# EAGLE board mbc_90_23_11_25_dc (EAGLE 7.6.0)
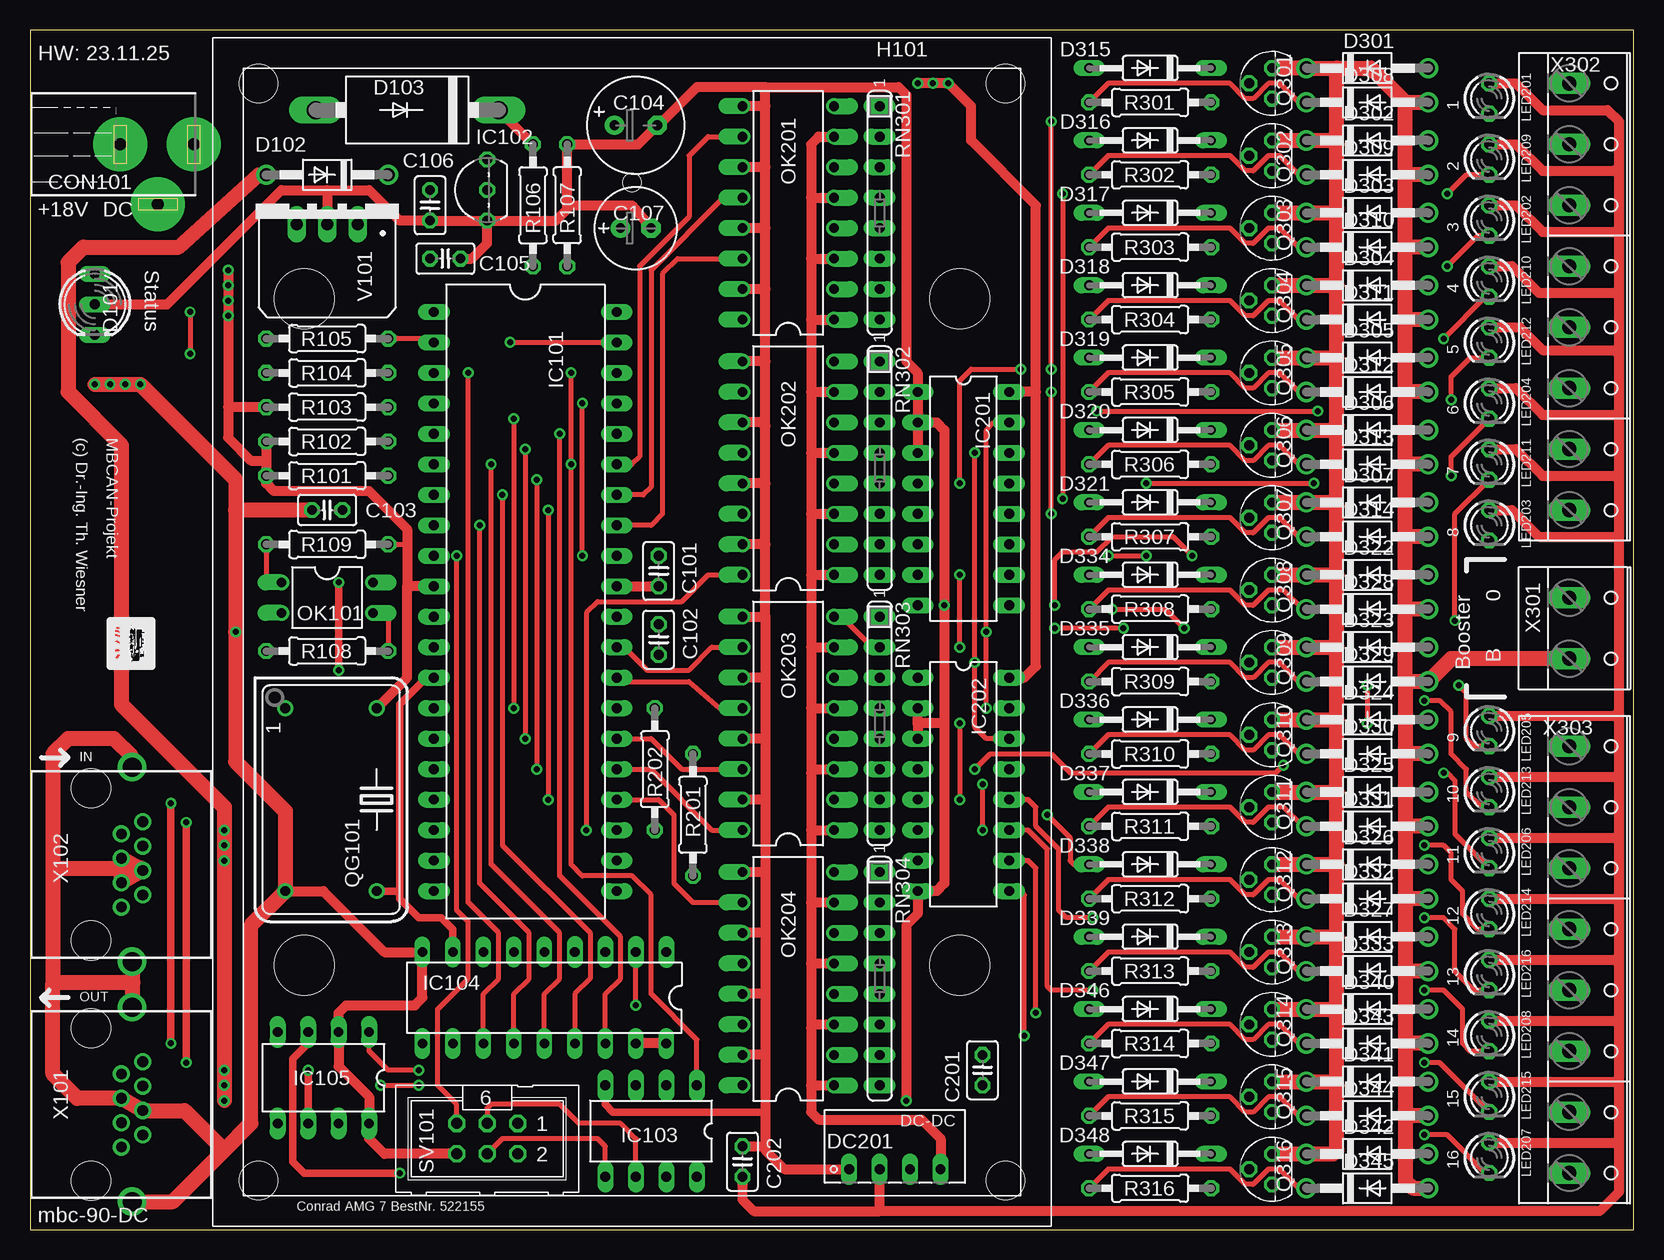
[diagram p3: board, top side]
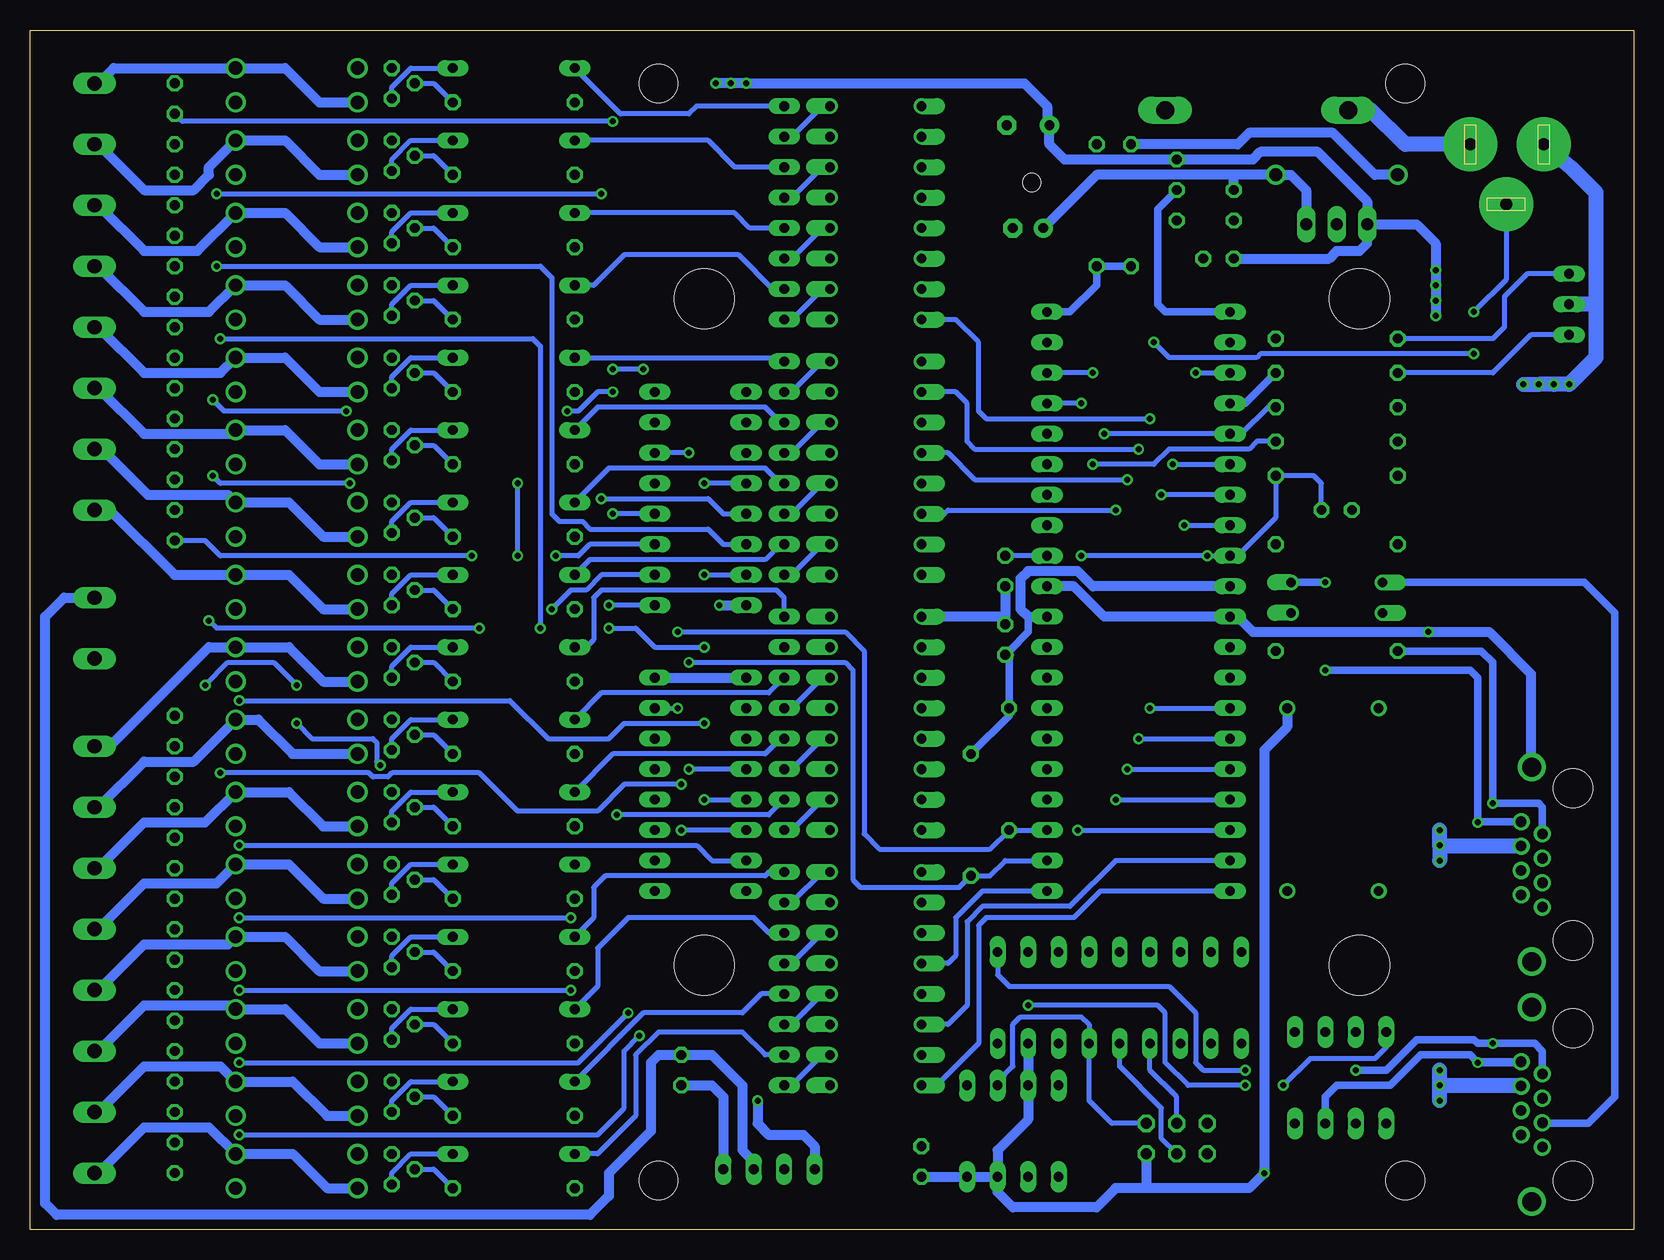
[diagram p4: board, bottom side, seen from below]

Size 133.66 x 99.99 mm. Coordinates in mm from the lower left corner, seen from the top.
Outline: 0,99.99 0,0 133.66,0 133.66,99.99 0,99.99
Copper layers (1*16): Top 0.035mm / dielectric 1.5mm / Bottom 0.035mm
Design rules "default *": minimum track width 10mil, minimum drill 0.5mm, track to track 8mil, track to pad 8mil, pad to pad 8mil, via to via 8mil, smd to smd 8mil, copper to edge 40mil, drill to drill 8mil, minimum pad ring 10mil, minimum via ring 8mil, stop-mask expansion 4mil, vias tented up to drill 0mil, thermal gap 10mil

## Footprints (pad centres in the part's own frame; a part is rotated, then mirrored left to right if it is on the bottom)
C025-025X050 = drill 0.813 octagon: 1 -1.27,0; 2 1.27,0
E3,5-8 = drill 0.813 pad 1.6: + -1.778,0 | drill 0.813 pad 1.6 octagon: - 1.778,0
E2,5-7 = drill 0.813 pad 1.6: + -1.27,0 | drill 0.813 pad 1.6 octagon: - 1.27,0
POWER-JACK = drill 1 pad 4.5: 1 0,6.03; 2 0,-0.12; 3 5,3.03
DUOLED5MM = drill 0.813 long: AG -2.54,0; AR 2.54,0; K 0,0
DO41-10 = drill 1.118: A 5.08,0; C -5.08,0
DO201-15 = drill 1.499 long: A 7.62,0; C -7.62,0
DO35-10 = drill 0.813 long: A 5.08,0; C -5.08,0
NME = drill 0.813 long: 1 0,3.81; 2 0,1.27; 3 0,-1.27; 4 0,-3.81
MODULGEHÄUSE-1 = hole 3.2: -45.72,-31.115; -45.72,31.115; 45.72,31.115; 45.72,-31.115 | hole 5: -27.781,-27.305; 27.781,-27.305; -27.781,27.305; 27.781,27.305 | hole 1.5: -37.465,0
DIL40 = drill 0.813 long: 1 -24.13,-7.62; 2 -21.59,-7.62; 3 -19.05,-7.62; 4 -16.51,-7.62; 5 -13.97,-7.62; 6 -11.43,-7.62; 7 -8.89,-7.62; 8 -6.35,-7.62; 9 -3.81,-7.62; 10 -1.27,-7.62; 11 1.27,-7.62; 12 3.81,-7.62; 13 6.35,-7.62; 14 8.89,-7.62; 15 11.43,-7.62; 16 13.97,-7.62; 17 16.51,-7.62; 18 19.05,-7.62; 19 21.59,-7.62; 20 24.13,-7.62; 21 24.13,7.62; 22 21.59,7.62; 23 19.05,7.62; 24 16.51,7.62; 25 13.97,7.62; 26 11.43,7.62; 27 8.89,7.62; 28 6.35,7.62; 29 3.81,7.62; 30 1.27,7.62; 31 -1.27,7.62; 32 -3.81,7.62; 33 -6.35,7.62; 34 -8.89,7.62; 35 -11.43,7.62; 36 -13.97,7.62; 37 -16.51,7.62; 38 -19.05,7.62; 39 -21.59,7.62; 40 -24.13,7.62
TO92- = drill 0.813 octagon: 1 -2.54,0; 2 0,0; 3 2.54,0
DIL8 = drill 0.813 long: 1 -3.81,-3.81; 2 -1.27,-3.81; 3 1.27,-3.81; 4 3.81,-3.81; 5 3.81,3.81; 6 1.27,3.81; 7 -1.27,3.81; 8 -3.81,3.81
DIL18 = drill 0.813 long: 1 -10.16,-3.81; 2 -7.62,-3.81; 3 -5.08,-3.81; 4 -2.54,-3.81 | drill 0.8 long: 5 0,-3.81; 6 2.54,-3.81; 7 5.08,-3.81; 8 7.62,-3.81; 9 10.16,-3.81; 10 10.16,3.81; 11 7.62,3.81; 12 5.08,3.81; 13 2.54,3.81; 14 0,3.81; 15 -2.54,3.81; 16 -5.08,3.81; 17 -7.62,3.81; 18 -10.16,3.81
DIL08 = drill 0.813 long: 1 -3.81,-3.81; 2 -1.27,-3.81; 3 1.27,-3.81; 4 3.81,-3.81; 5 3.81,3.81; 6 1.27,3.81; 7 -1.27,3.81; 8 -3.81,3.81
DIL16 = drill 0.813 long: 1 -8.89,-3.81; 2 -6.35,-3.81; 3 -3.81,-3.81; 4 -1.27,-3.81; 5 1.27,-3.81; 6 3.81,-3.81; 7 6.35,-3.81; 8 8.89,-3.81; 9 8.89,3.81; 10 6.35,3.81; 11 3.81,3.81; 12 1.27,3.81; 13 -1.27,3.81; 14 -3.81,3.81; 15 -6.35,3.81; 16 -8.89,3.81
LED3MM = drill 0.813 octagon: A -1.27,0; K 1.27,0
DIL04 = drill 0.813 offset: 1 -1.27,-3.81; 2 1.27,-3.81; 3 1.27,3.81; 4 -1.27,3.81
DIL16' = drill 0.813 offset: 1 -8.89,-3.81; 2 -6.35,-3.81; 3 -3.81,-3.81; 4 -1.27,-3.81; 5 1.27,-3.81; 6 3.81,-3.81; 7 6.35,-3.81; 8 8.89,-3.81; 9 8.89,3.81; 10 6.35,3.81; 11 3.81,3.81; 12 1.27,3.81; 13 -1.27,3.81; 14 -3.81,3.81; 15 -6.35,3.81; 16 -8.89,3.81
TO92 = drill 0.813 octagon: 1 1.27,0; 2 0,1.905; 3 -1.27,0
DIL14S = drill 0.813: 1 -7.62,-3.81; 7 7.62,-3.81; 8 7.62,3.81; 14 -7.62,3.81
0207/10 = drill 0.813 octagon: 1 -5.08,0; 2 5.08,0
SIL8 = drill 0.813 long: 1 -8.89,0; 2 -6.35,0; 3 -3.81,0; 4 -1.27,0; 5 1.27,0; 6 3.81,0; 7 6.35,0; 8 8.89,0
ML6 = drill 0.914 octagon: 1 -2.54,-1.27; 2 -2.54,1.27; 3 0,-1.27; 4 0,1.27; 5 2.54,-1.27; 6 2.54,1.27
TRACO-TSR-1 = drill 1.016 long: GND 0,2.54; IN -2.54,2.54; OUT 2.54,2.54
0446200002 = drill 0.889 pad 1.422: 1 3.556,2.54; 2 2.54,4.318; 3 1.524,2.54; 4 0.508,4.318; 5 -0.508,2.54; 6 -1.524,4.318; 7 -2.54,2.54; 8 -3.556,4.318 | drill 1.575 pad 2.286: S@1 -8.103,3.429; S@2 8.103,3.429 | hole 3.251: 6.35,0; -6.35,0
W237-132 = drill 1.194 long: 1 -2.54,-0.635; 2 2.54,-0.635
W237-8P = drill 1.194 long: 1 -17.78,-0.635; 2 -12.7,-0.635; 3 -7.62,-0.635; 4 -2.54,-0.635; 5 2.54,-0.635; 6 7.62,-0.635; 7 12.7,-0.635; 8 17.78,-0.635

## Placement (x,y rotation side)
C101  100n  [C025-025X050]  52.39,54.91 270 top
C102  100n  [C025-025X050]  52.39,49.19 90 top
C103  100n  [C025-025X050]  24.77,59.99 180 top
C104  470u/16V  [E3,5-8]  50.48,92.06 0 top
C105  100n  [C025-025X050]  34.61,80.94 0 top
C106  100n  [C025-025X050]  33.34,85.39 270 top
C107  47u/35V  [E2,5-7]  50.48,83.48 0 top
C201  100n  [C025-025X050]  79.38,13.32 90 top
C202  100n  [C025-025X050]  59.37,5.7 90 top
CON101  [POWER-JACK]  7.62,90.47 270 top
D101  Status  [DUOLED5MM]  5.4,77.13 270 top
D102  1N4004  [DO41-10]  24.77,87.93 180 top
D103  1N5400  [DO201-15]  31.43,93.33 180 top
D301  1N4001  [DO41-10]  111.44,96.82 0 top
D302  1N4001  [DO41-10]  111.44,90.79 0 top
D303  1N4001  [DO41-10]  111.44,84.75 0 top
D304  1N4001  [DO41-10]  111.44,78.72 0 top
D305  1N4001  [DO41-10]  111.44,72.69 0 top
D306  1N4001  [DO41-10]  111.44,66.66 0 top
D307  1N4001  [DO41-10]  111.44,60.62 0 top
D308  1N4001  [DO41-10]  111.44,93.96 0 top
D309  1N4001  [DO41-10]  111.44,87.93 0 top
D310  1N4001  [DO41-10]  111.44,81.9 0 top
D311  1N4001  [DO41-10]  111.44,75.86 0 top
D312  1N4001  [DO41-10]  111.44,69.83 0 top
D313  1N4001  [DO41-10]  111.44,63.8 0 top
D314  1N4001  [DO41-10]  111.44,57.76 0 top
D315  1N4148  [DO35-10]  93.34,96.82 180 top
D316  1N4148  [DO35-10]  93.34,90.79 180 top
D317  1N4148  [DO35-10]  93.34,84.75 180 top
D318  1N4148  [DO35-10]  93.34,78.72 180 top
D319  1N4148  [DO35-10]  93.34,72.69 180 top
D320  1N4148  [DO35-10]  93.34,66.66 180 top
D321  1N4148  [DO35-10]  93.34,60.62 180 top
D322  1N4001  [DO41-10]  111.44,54.59 0 top
D323  1N4001  [DO41-10]  111.44,48.56 0 top
D324  1N4001  [DO41-10]  111.44,42.52 0 top
D325  1N4001  [DO41-10]  111.44,36.49 0 top
D326  1N4001  [DO41-10]  111.44,30.46 0 top
D327  1N4001  [DO41-10]  111.44,24.43 0 top
D328  1N4001  [DO41-10]  111.44,51.73 0 top
D329  1N4001  [DO41-10]  111.44,45.7 0 top
D330  1N4001  [DO41-10]  111.44,39.67 0 top
D331  1N4001  [DO41-10]  111.44,33.63 0 top
D332  1N4001  [DO41-10]  111.44,27.6 0 top
D333  1N4001  [DO41-10]  111.44,21.57 0 top
D334  1N4148  [DO35-10]  93.34,54.59 180 top
D335  1N4148  [DO35-10]  93.34,48.56 180 top
D336  1N4148  [DO35-10]  93.34,42.52 180 top
D337  1N4148  [DO35-10]  93.34,36.49 180 top
D338  1N4148  [DO35-10]  93.34,30.46 180 top
D339  1N4148  [DO35-10]  93.34,24.43 180 top
D340  1N4001  [DO41-10]  111.44,18.39 0 top
D341  1N4001  [DO41-10]  111.44,12.36 0 top
D342  1N4001  [DO41-10]  111.44,6.33 0 top
D343  1N4001  [DO41-10]  111.44,15.54 0 top
D344  1N4001  [DO41-10]  111.44,9.51 0 top
D345  1N4001  [DO41-10]  111.44,3.47 0 top
D346  1N4148  [DO35-10]  93.34,18.39 180 top
D347  1N4148  [DO35-10]  93.34,12.36 180 top
D348  1N4148  [DO35-10]  93.34,6.33 180 top
DC201  NKE0505  [NME]  72.07,5.06 90 top
H101  [MODULGEHÄUSE-1]  50.16,49.83 270 top
IC101  MEGA644-P  [DIL40]  41.27,52.37 270 top
IC102  DS1820  [TO92-]  38.1,86.66 90 top
IC103  25LC10240P  [DIL8]  51.75,8.24 180 top
IC104  MCP2515-I/P  [DIL18]  42.86,19.35 180 top
IC105  PCA82C250  [DIL08]  24.45,12.68 180 top
IC201  PCF8574P  [DIL16]  77.79,60.94 270 top
IC202  PCF8574P  [DIL16]  77.79,37.13 270 top
LED201  Gelb 5V 3mm  [LED3MM]  121.6,94.28 270 top
LED202  Gelb 5V 3mm  [LED3MM]  121.6,84.12 270 top
LED203  Gelb 5V 3mm  [LED3MM]  121.6,58.72 270 top
LED204  Gelb 5V 3mm  [LED3MM]  121.6,68.88 270 top
LED205  Gelb 5V 3mm  [LED3MM]  121.6,41.57 270 top
LED206  Gelb 5V 3mm  [LED3MM]  121.6,31.41 270 top
LED207  Gelb 5V 3mm  [LED3MM]  121.6,6.01 270 top
LED208  Gelb 5V 3mm  [LED3MM]  121.6,16.17 270 top
LED209  Gelb 5V 3mm  [LED3MM]  121.6,89.2 270 top
LED210  Gelb 5V 3mm  [LED3MM]  121.6,79.04 270 top
LED211  Gelb 5V 3mm  [LED3MM]  121.6,63.8 270 top
LED212  Gelb 5V 3mm  [LED3MM]  121.6,73.96 270 top
LED213  Gelb 5V 3mm  [LED3MM]  121.6,36.49 270 top
LED214  Gelb 5V 3mm  [LED3MM]  121.6,26.33 270 top
LED215  Gelb 5V 3mm  [LED3MM]  121.6,11.09 270 top
LED216  Gelb 5V 3mm  [LED3MM]  121.6,21.25 270 top
OK101  PC814  [DIL04]  24.77,52.68 270 top
OK201  PC 847X  [DIL16']  63.18,84.75 90 top
OK202  PC 847X  [DIL16']  63.18,63.48 90 top
OK203  PC 847X  [DIL16']  63.18,42.21 90 top
OK204  PC 847X  [DIL16']  63.18,20.93 90 top
Q301  BC547A  [TO92]  103.5,95.55 90 top
Q302  BC547A  [TO92]  103.5,89.52 90 top
Q303  BC547A  [TO92]  103.5,83.48 90 top
Q304  BC547A  [TO92]  103.5,77.45 90 top
Q305  BC547A  [TO92]  103.5,71.42 90 top
Q306  BC547A  [TO92]  103.5,65.39 90 top
Q307  BC547A  [TO92]  103.5,59.35 90 top
Q308  BC547A  [TO92]  103.5,53.32 90 top
Q309  BC547A  [TO92]  103.5,47.29 90 top
Q310  BC547A  [TO92]  103.5,41.25 90 top
Q311  BC547A  [TO92]  103.5,35.22 90 top
Q312  BC547A  [TO92]  103.5,29.19 90 top
Q313  BC547A  [TO92]  103.5,23.16 90 top
Q314  BC547A  [TO92]  103.5,17.12 90 top
Q315  BC547A  [TO92]  103.5,11.09 90 top
Q316  BC547A  [TO92]  103.5,5.06 90 top
QG101  16 MHz  [DIL14S]  25.08,35.86 270 top
R101  10k  [0207/10]  24.77,62.84 180 top
R102  10k  [0207/10]  24.77,65.7 180 top
R103  10k  [0207/10]  24.77,68.56 180 top
R104  390R  [0207/10]  24.77,71.42 180 top
R105  390R  [0207/10]  24.77,74.28 180 top
R106  9k/0,1%  [0207/10]  41.91,85.39 270 top
R107  1k/0,1%  [0207/10]  44.77,85.39 90 top
R108  120R  [0207/10]  24.77,48.24 180 top
R109  390R  [0207/10]  24.77,57.13 180 top
R201  4k7  [0207/10]  55.24,34.59 90 top
R202  4k7  [0207/10]  52.07,38.4 90 top
R301  1k  [0207/10]  93.34,93.96 0 top
R302  1k  [0207/10]  93.34,87.93 0 top
R303  1k  [0207/10]  93.34,81.9 0 top
R304  1k  [0207/10]  93.34,75.86 0 top
R305  1k  [0207/10]  93.34,69.83 0 top
R306  1k  [0207/10]  93.34,63.8 0 top
R307  1k  [0207/10]  93.34,57.76 0 top
R308  1k  [0207/10]  93.34,51.73 0 top
R309  1k  [0207/10]  93.34,45.7 0 top
R310  1k  [0207/10]  93.34,39.67 0 top
R311  1k  [0207/10]  93.34,33.63 0 top
R312  1k  [0207/10]  93.34,27.6 0 top
R313  1k  [0207/10]  93.34,21.57 0 top
R314  1k  [0207/10]  93.34,15.54 0 top
R315  1k  [0207/10]  93.34,9.51 0 top
R316  1k  [0207/10]  93.34,3.47 0 top
RN301  10k  [SIL8]  70.8,84.75 270 top
RN302  10k  [SIL8]  70.8,63.48 270 top
RN303  10k  [SIL8]  70.8,42.21 270 top
RN304  10k  [SIL8]  70.8,20.93 270 top
SV101  [ML6]  38.1,7.6 180 top
V101  TSR-1  [TRACO-TSR-1]  24.77,86.34 180 top
X101  OUT  [0446200002]  5.08,10.46 270 top
X102  IN  [0446200002]  5.08,30.46 270 top
X301  [W237-132]  128.91,50.14 270 top
X302  [W237-8P]  128.91,77.77 270 top
X303  [W237-8P]  128.91,22.52 270 top

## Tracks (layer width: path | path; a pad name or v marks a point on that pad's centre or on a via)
1-WIRE
  Bottom 0.61: IC102.2 39.69,85.07 39.69,77.13 39.05,76.5 IC101.1
+5V  (via drill 0.5)
  Top 0.406: R109.1 31.43,57.13
  Top 0.61: IC105.3 23.18,15.54 21.91,14.27 21.91,5.7 22.86,4.74 v30.8,4.74
  Top 0.813: IC104.18 IC104.17 | 31.43,53.64 31.43,57.13 31.43,58.4 28.26,61.57 20.32,61.57 19.68,62.21 R101.2 19.68,64.12 | v16.51,79.99 v16.51,78.72 v16.51,77.45 v16.51,76.18 16.51,68.56 | 16.51,68.56 16.51,66.02 18.41,64.12 19.68,64.12 | IC101.10 31.43,53.64 | QG101.14 31.43,46.02 31.43,53.64 | R103.2 16.51,68.56 | R102.2 19.68,64.12 | LED201.A 123.83,95.55 126.05,93.33 131.44,93.33 132.4,92.37 132.4,88.56 | 132.4,88.56 132.4,83.17 | 132.4,83.17 132.4,77.77 | 132.4,77.77 132.4,73.01 | 132.4,73.01 132.4,67.92 | 132.4,67.92 132.4,62.53 | 132.4,62.53 132.4,57.76 | 132.4,57.76 132.4,43.16 | 132.4,43.16 132.4,37.76 | 132.4,37.76 132.4,32.68 | 132.4,32.68 132.4,27.6 | 132.4,27.6 132.4,22.21 | 132.4,22.21 132.4,17.44 | 132.4,17.44 132.4,12.36 | 132.4,12.36 132.4,7.28 | 132.4,7.28 132.4,3.15 130.81,1.57 70.8,1.57 | 70.8,1.57 DC201.2 | C202.1 59.37,2.52 60.33,1.57 70.8,1.57 | LED207.A 132.4,7.28 | LED215.A 132.4,12.36 | LED208.A 132.4,17.44 | LED216.A 132.08,22.52 132.4,22.21 | LED214.A 132.4,27.6 | LED206.A 132.4,32.68 | LED213.A 132.4,37.76 | LED205.A 132.08,42.84 132.4,43.16 | LED203.A 123.51,59.99 125.73,57.76 132.4,57.76 | LED211.A 123.83,65.07 126.05,62.84 132.08,62.84 132.4,62.53 | LED204.A 123.83,70.15 126.05,67.92 132.4,67.92 | LED212.A 124.14,75.23 126.05,73.32 132.08,73.32 132.4,73.01 | LED210.A 123.51,80.31 125.73,78.09 132.08,78.09 132.4,77.77 | LED202.A 123.83,85.39 126.05,83.17 132.4,83.17 | LED209.A 123.83,90.47 126.05,88.25 132.08,88.25 132.4,88.56 | IC202.16 82.87,46.02 83.82,46.97 83.82,69.83 | 83.82,69.83 IC201.16 | 83.82,69.83 83.82,85.39 78.42,90.79 78.42,93.64 v76.52,95.55 v75.25,95.55 v73.98,95.55
  Bottom 0.406: 48.9,92.06 C104.+
  Bottom 0.61: 50.48,51.1 50.48,49.83 52.07,48.24 52.07,47.92 R202.2 52.07,42.84 R201.2
  Bottom 0.813: V101.OUT 18.1,83.8 16.51,82.21 v16.51,79.99 v16.51,78.72 v16.51,77.45 v16.51,76.18 | QG101.14 28.89,41.89 30.8,39.98 v30.8,4.74 32.07,3.47 40.64,3.47 | IC101.10 45.09,53.64 46.35,54.91 50.48,54.91 51.12,54.27 51.12,51.73 50.48,51.1 IC101.30 | V101.OUT 22.23,85.7 26.35,89.83 31.11,89.83 31.75,89.2 IC102.3 47.43,89.2 48.7,90.47 C104.+ | IC202.16 IC202.1 | IC104.17 IC103.3 50.48,9.19 53.02,6.65 IC103.7 | C202.1 IC103.8 IC103.7 | 40.64,3.47 43.18,3.47 44.77,1.89 51.75,1.89 53.02,3.15 IC103.7 | SV101.2 40.64,3.47 | C105.1 25.4,80.94 24.77,81.58 22.86,81.58 22.23,82.21 V101.OUT | C102.1 52.07,47.92 | 48.9,92.06 48.9,93.64 50.8,95.55 v73.98,95.55 v76.52,95.55
+18V  (via drill 0.5)
  Top 0.813: R106.1 D103.C
  Top 1.27: D102.A 19.05,87.93 12.38,81.9 4.45,81.9 3.17,80.62 3.17,69.83 7.62,65.39 7.62,43.79 16.19,35.22 v16.19,33.32 v16.19,32.05 v16.19,30.78 v16.19,13.32 v16.19,12.04 v16.19,10.78
  Bottom 0.813: R106.1 33.02,90.47 32.07,91.42 25.08,91.42 21.59,87.93 D102.A
  Bottom 1.27: v16.19,12.04 9.46,12.04 X101.6 | v16.19,10.78 v16.19,12.04 | v16.19,12.04 v16.19,13.32 | X102.6 16.13,31.98 v16.19,32.05 | v16.19,32.05 v16.19,33.32 | v16.19,32.05 v16.19,30.78
/CS-MBC  (via drill 0.5)
  Top 0.406: IC104.16 47.94,19.66 49.21,20.93 49.21,24.43 44.13,29.51 v44.13,66.34
  Bottom 0.406: R103.1 30.48,68.56 32.7,66.34 IC101.5 v44.13,66.34
/CS-MEM  (via drill 0.5)
  Top 0.406: IC103.1 55.56,15.86 51.75,19.66 51.75,27.92 50.16,29.51 46.04,29.51 45.09,30.46 v45.09,63.8 v45.09,71.42
  Bottom 0.406: v45.09,71.42 IC101.38 | R102.1 31.43,65.7 32.07,65.07 38.73,65.07 40.01,63.8 v45.09,63.8
/INT  (via drill 0.5)
  Top 0.406: IC104.12 37.78,19.66 39.05,20.93 39.05,24.75 36.51,27.29 v36.51,71.42
  Bottom 0.406: v36.51,71.42 IC101.3
/RES  (via drill 0.5)
  Top 0.406: SV101.5 35.56,10.46 33.97,12.04 33.97,18.39 36.51,20.93 36.51,25.7 35.56,26.65 v35.56,56.18 | v46.04,56.18 v46.04,68.88
  Bottom 0.406: C103.1 26.04,62.21 26.67,62.84 R101.1 29.84,59.35 33.02,56.18 IC101.9 v35.56,56.18 v46.04,56.18 | v46.04,68.88 IC101.37
AREF
  Bottom 0.406: IC101.32 C101.1
CAN-H  (via drill 0.5)
  Top 0.61: v13.02,13.95 v13.02,33.95 | v25.72,46.65 v25.72,53.95
  Bottom 0.61: IC105.7 25.72,11.09 24.77,12.04 20.32,12.04 17.78,14.59 13.65,14.59 13.08,14.01 X101.8 9.46,14.01 9.53,13.95 v13.02,13.95 | v13.02,33.95 13.02,34.02 | 13.02,34.02 X102.8 | 13.02,34.02 13.02,46.02 13.65,46.65 v25.72,46.65 | v25.72,53.95 OK101.4
CAN-L  (via drill 0.5)
  Top 0.61: v23.18,13.32 IC105.6 | v11.75,15.54 v11.75,35.54
  Bottom 0.61: X101.7 7.62,14.9 8.26,15.54 v11.75,15.54 13.02,15.54 13.34,15.86 18.1,15.86 20.64,13.32 v23.18,13.32 | X102.7 7.62,35.22 7.94,35.54 v11.75,35.54 11.75,47.29 12.7,48.24 R108.2
GND  (via drill 0.5)
  Top 0.406: 52.39,92.06 C104.-
  Top 0.61: IC103.4 47.94,10.46 48.58,9.82 61.28,9.82
  Top 0.813: IC101.31 C101.2 | C104.- 50.67,90.47 R107.2 44.77,85.39 | 44.77,85.39 44.77,85.07 43.81,84.12 IC102.1 | 24.77,86.66 V101.GND | 24.77,86.66 28.26,86.66 30.8,84.12 C106.2 IC102.1 | D101.K 11.43,77.13 20.95,86.66 24.77,86.66 | 73.98,42.21 IC202.2 | 73.98,42.21 IC202.3 | IC201.2 IC201.3 | 61.28,93.64 OK201.9 | 61.28,88.56 61.28,93.64 | 61.28,83.48 61.28,88.56 | 61.28,78.4 61.28,83.48 | 61.28,72.37 61.28,78.4 | 61.28,66.97 61.28,72.37 | 61.28,62.21 61.28,66.97 | 61.28,57.13 61.28,62.21 | 61.28,51.1 61.28,57.13 | 61.28,51.1 61.28,46.02 | 61.28,46.02 61.28,40.94 | 61.28,40.94 61.28,35.86 | 61.28,24.75 61.28,19.66 | 61.28,19.66 61.28,14.59 | 61.28,14.59 OK204.15 | 61.28,19.66 OK204.13 | 61.28,24.75 OK204.11 | 61.28,29.82 OK204.9 | 61.28,29.82 61.28,24.75 | 61.28,35.86 OK203.15 | 61.28,35.86 61.28,29.82 | 61.28,40.94 OK203.13 | 61.28,46.02 OK203.11 | OK203.9 61.28,51.1 | 61.28,88.56 OK201.11 | 61.28,83.48 OK201.13 | 61.28,78.4 OK201.15 | 61.28,72.37 OK202.9 | OK202.11 60.96,67.29 61.28,66.97 | 61.28,62.21 OK202.13 | 61.28,57.13 OK202.15 | IC201.2 IC201.1 73.98,71.42 73.03,72.37 73.03,94.59 72.39,95.23 61.28,95.23 | 76.2,42.21 v76.2,52.05 76.2,66.66 75.56,67.29 IC201.2 | 76.2,42.21 73.98,42.21 | 61.28,93.64 61.28,95.23 | 61.28,95.23 55.56,95.23 52.39,92.06 | 76.2,42.21 76.2,28.87 75.56,28.24 IC202.8 73.98,26.33 73.03,25.38 v73.03,10.78 | C107.- 50.16,85.39 44.77,85.39 | 61.28,14.59 61.28,9.82 61.28,6.97 | 61.28,6.97 61.28,6.65 62.87,5.06 DC201.1 | SV101.6 29.53,6.33 28.26,7.6 IC105.8 28.26,11.09 25.72,13.63 IC105.2 25.72,18.08 26.35,18.71 32.07,18.71 32.7,19.35 IC104.9 29.53,23.16 24.45,28.24 QG101.7 | C105.2 36.83,80.94 38.1,82.21 IC102.1
  Top 0.813: C202.2 61.28,6.97
  Top 1.27: v5.4,70.47 v9.21,70.47 17.14,62.53 17.14,59.99 | 17.14,59.99 v17.14,49.83 17.14,39.03 21.27,34.9 QG101.7 18.41,25.38 18.41,8.87 16.19,6.65 | C103.2 17.14,59.99 | X101.S@2 11.9,2.35 16.19,6.65 | 16.19,6.65 12.89,9.95 X101.4 X101.5 3.94,10.97 1.91,13 1.91,20.62 | X102.4 X102.3 7.62,30.14 | X102.4 X102.5 | X101.S@1 X102.S@2 8.51,20.68 8.57,20.62 1.91,20.62 | 1.91,30.14 7.62,30.14 | 7.62,30.14 9.21,30.14 X102.4 | X102.S@1 8.51,39.41 6.99,40.94 3.17,40.94 1.91,39.67 1.91,30.14 | 1.91,30.14 1.91,20.62
  Bottom 0.813: IC101.31 46.67,53.64 44.13,51.1 IC101.11 33.02,51.1 31.75,49.83 v17.14,49.83 12.06,49.83 8.57,46.33 8.57,38.4 | v76.2,52.05 IC201.8 | 52.39,51.1 OK203.9 | C101.2 52.39,51.1 | v73.03,10.78 73.03,8.87 72.07,7.92 69.22,7.92 68.26,6.97 DC201.1 | C102.2 52.39,51.1
  Bottom 1.27: 3.17,77.13 3.17,86.46 5.28,88.56 CON101.2 | 3.17,77.13 D101.K | 3.17,77.13 3.17,72.69 v5.4,70.47 v6.67,70.47 v7.94,70.47 v9.21,70.47
GNDA
  Bottom 0.813: DC201.3 73.34,5.7 74.3,6.65 74.3,12.04 76.83,14.59 C201.2 81.28,14.59 81.92,13.95 81.92,8.24 85.41,4.74 85.41,2.84 87,1.25 131.44,1.25 132.4,2.2 132.4,51.1 130.81,52.68 X301.1
I00
  Top 0.406: IC101.35 50.16,63.8 50.8,64.43 50.8,80.31 54.93,84.44 54.93,89.52 56.52,91.1 OK201.10
I01
  Top 0.406: IC101.34 51.12,61.26 51.75,61.89 51.75,79.99 57.78,86.02 OK201.12
I02
  Top 0.406: IC101.33 51.75,58.72 52.7,59.67 52.7,79.67 53.98,80.94 OK201.14
I03  (via drill 0.5)
  Top 0.406: v40.32,67.61 v40.32,43.48
  Bottom 0.406: v40.32,43.48 IC101.14 | v40.32,67.61 53.98,67.61 54.61,68.24 54.61,73.96 56.52,75.86 OK201.16
I04  (via drill 0.5)
  Top 0.406: v41.27,65.07 v41.27,40.94
  Bottom 0.406: v41.27,40.94 IC101.15 | v41.27,65.07 54.93,65.07 55.56,65.7 55.56,68.88 56.52,69.83 OK202.10
I05  (via drill 0.5)
  Top 0.406: v42.23,62.53 v42.23,38.4
  Bottom 0.406: v42.23,38.4 IC101.16 | v42.23,62.53 54.93,62.53 57.15,64.75 OK202.12
I06  (via drill 0.5)
  Top 0.406: v43.18,59.99 v43.18,35.86
  Bottom 0.406: v43.18,35.86 IC101.17 | v43.18,59.99 57.15,59.99 57.47,59.67 OK202.14
I07  (via drill 0.5)
  Top 0.406: v46.35,33.32 46.35,51.41 47.31,52.37 54.29,52.37 56.52,54.59 OK202.16
  Bottom 0.406: v46.35,33.32 IC101.18
I08
  Top 0.406: IC101.29 49.53,48.56 51.44,46.65 54.93,46.65 56.83,48.56 OK203.10
I09
  Top 0.406: IC101.28 49.21,46.02 49.53,45.7 54.93,45.7 57.47,43.48 OK203.12
I10
  Top 0.406: IC101.26 51.75,40.94 54.29,38.4 OK203.14
I11
  Top 0.406: IC101.25 51.75,38.4 56.83,33.32 OK203.16
I12
  Top 0.406: IC101.24 52.39,35.86 53.66,34.59 53.66,28.87 55.24,27.29 OK204.10
I13
  Bottom 0.406: IC101.21 54.29,28.24 56.52,26.02 56.52,22.84 57.15,22.21 OK204.12
I14
  Bottom 0.406: IC101.19 43.18,30.78 46.99,26.97 54.29,26.97 55.56,25.7 55.56,18.71 57.15,17.12 OK204.14
I15
  Bottom 0.406: IC101.20 44.45,28.24 46.67,26.02 53.98,26.02 54.61,25.38 54.61,15.54 58.1,12.04 OK204.16
IN
  Top 1.27: X301.2 118.43,47.6 D329.A 114.62,45.7 | 114.62,45.7 114.62,51.73 | 114.62,51.73 114.62,57.76 | 114.62,57.76 114.62,63.8 | 114.62,63.8 114.62,69.51 | 114.62,69.51 114.62,75.86 | 114.62,75.86 114.62,81.9 | 114.62,81.9 114.62,87.93 | 114.62,87.93 114.62,93.96 | 114.62,93.96 D308.A | 108.9,96.82 D301.C Q301.1 | 108.9,96.82 111.76,96.82 114.62,93.96 | D309.A 114.62,87.93 | D310.A 114.62,81.9 | D311.A 114.62,75.86 | D312.A 114.94,69.83 114.62,69.51 | D313.A 114.62,63.8 | D314.A 114.62,57.76 | D328.A 114.62,51.73 | 114.62,45.7 114.62,39.67 | 114.62,39.67 114.62,33.63 | D330.A 114.62,39.67 | D331.A 114.62,33.63 | 114.62,33.63 114.62,27.6 | 114.62,27.6 114.62,21.57 | 114.62,21.57 114.62,15.54 | 114.62,15.54 114.62,9.51 | 114.62,9.51 114.62,4.11 115.25,3.47 D345.A | D344.A 114.62,9.51 | D343.A 114.62,15.54 | D333.A 114.62,21.57 | D332.A 114.62,27.6 | Q302.1 D302.C 108.58,90.79 108.9,90.47 | Q303.1 D303.C 108.58,84.75 108.9,85.07 | Q304.1 D304.C 108.9,78.72 | Q305.1 D305.C 108.9,72.69 | Q306.1 D306.C 108.58,66.66 108.9,66.97 | Q307.1 D307.C 108.58,60.62 108.9,60.3 | Q308.1 D322.C 108.9,54.59 | Q309.1 D323.C 108.9,48.56 | Q310.1 D324.C 108.9,42.52 | Q311.1 D325.C 108.9,36.49 | Q312.1 D326.C 108.9,30.46 | Q313.1 D327.C 108.9,24.43 | Q314.1 D340.C 108.9,18.39 | D341.C Q315.1 108.58,12.36 108.9,12.04 | Q316.1 D342.C 108.58,6.33 108.9,6.65 108.9,12.04 | 108.9,12.04 108.9,18.39 | 108.9,18.39 108.9,24.43 | 108.9,24.43 108.9,30.46 | 108.9,30.46 108.9,36.49 | 108.9,36.49 108.9,42.52 | 108.9,42.52 108.9,48.56 | 108.9,48.56 108.9,54.59 | 108.9,54.59 108.9,60.3 | 108.9,60.3 108.9,66.97 | 108.9,66.97 108.9,72.69 | 108.9,72.69 108.9,78.72 | 108.9,78.72 108.9,85.07 | 108.9,85.07 108.9,90.47
  Top 1.27: 108.9,90.47 108.9,96.82
IN0
  Bottom 0.406: OK201.8 67.63,93.64 70.17,91.1 RN301.2
IN1
  Bottom 0.406: OK201.6 67.63,88.56 70.17,86.02 RN301.4
IN2
  Bottom 0.406: OK201.4 67.63,83.48 70.17,80.94 RN301.6
IN3
  Bottom 0.406: OK201.2 67.63,78.4 70.17,75.86 RN301.8
IN4
  Bottom 0.406: OK202.8 67.63,72.37 70.17,69.83 RN302.2
IN5
  Bottom 0.406: OK202.6 67.63,67.29 70.17,64.75 RN302.4
IN6
  Bottom 0.406: OK202.4 67.63,62.21 70.17,59.67 RN302.6
IN7
  Bottom 0.406: OK202.2 67.63,57.13 70.17,54.59 RN302.8
IN8
  Top 0.406: OK203.8 67.63,51.1 70.17,48.56 RN303.2
IN9
  Bottom 0.406: OK203.6 67.63,46.02 70.17,43.48 RN303.4
IN10
  Bottom 0.406: OK203.4 67.63,40.94 70.17,38.4 RN303.6
IN11
  Bottom 0.406: OK203.2 67.63,35.86 70.17,33.32 RN303.8
IN12
  Bottom 0.406: OK204.8 67.63,29.82 70.17,27.29 RN304.2
IN13
  Bottom 0.406: OK204.6 67.63,24.75 70.17,22.21 RN304.4
IN14
  Bottom 0.406: OK204.4 67.63,19.66 70.17,17.12 RN304.6
IN15
  Bottom 0.406: OK204.2 67.63,14.59 70.17,12.04 RN304.8
LED-G
  Top 0.406: IC101.2 32.7,74.28 R105.1
LED-R
  Bottom 0.61: IC101.4 32.38,68.88 R104.1
MISO  (via drill 0.5)
  Top 0.406: v39.37,61.26 39.37,32.05 46.67,24.75 46.67,20.93 45.4,19.66 IC104.15
  Bottom 0.406: SV101.1 43.5,8.87 45.4,10.78 IC104.15 45.4,17.12 46.04,17.76 51.12,17.76 51.75,17.12 51.75,13.63 53.02,12.36 IC103.2 | IC101.7 v39.37,61.26
MOSI  (via drill 0.5)
  Top 0.406: IC103.5 47.94,6.97 47.31,7.6 39.37,7.6 SV101.4 | IC104.14 42.86,19.66 44.13,20.93 44.13,24.75 38.42,30.46 v38.42,63.8
  Bottom 0.406: SV101.4 39.37,7.6 39.37,10.14 42.86,13.63 IC104.14 | v38.42,63.8 IC101.6
N$1  (via drill 0.5)
  Top 0.406: v32.38,13.32 29.84,13.32 28.26,14.9 IC105.1
  Bottom 0.406: IC104.1 53.02,21.25 52.07,20.3 38.73,20.3 36.51,18.08 36.51,13.95 35.88,13.32 v32.38,13.32
N$2  (via drill 0.5)
  Top 0.406: v29.21,12.04 v32.38,12.04 | v50.48,18.71 IC104.2
  Bottom 0.406: IC105.4 20.64,15.22 21.59,14.27 26.99,14.27 v29.21,12.04 | v32.38,12.04 37.15,12.04 39.05,13.95 39.05,18.08 39.69,18.71 v50.48,18.71
N$3
  Bottom 0.406: Q302.2 100.01,89.52 R302.2
N$4
  Top 0.406: OK101.3 29.84,51.41 R108.1
N$5
  Bottom 0.406: Q302.3 103.5,89.2 101.92,90.79 D316.C
N$6
  Bottom 0.813: C107.+ 44.77,87.93 33.34,87.93 | 33.34,87.93 D102.C 28.57,87.93 27.3,86.66 V101.IN | C106.1 33.34,87.93
N$7
  Top 0.406: R109.2 19.68,53.95 OK101.1
  Bottom 0.61: OK101.1 4.13,53.95 1.59,51.41 1.59,11.09 3.81,8.87 7.56,8.87 X101.3
N$8
  Bottom 0.406: RN301.3 74.93,88.56 77.15,90.79 D316.A
N$9
  Bottom 0.406: D101.AR 8.57,74.59 11.75,71.42 R104.2
N$10
  Bottom 0.406: Q303.2 100.01,83.48 R303.2
N$11
  Bottom 0.406: Q303.3 103.5,83.17 101.92,84.75 D317.C
N$12
  Bottom 0.406: RN301.5 73.66,83.48 74.93,84.75 D317.A
N$13
  Bottom 0.406: D101.AG 8.89,79.67 10.79,77.77 10.79,75.23 11.75,74.28 R105.2
N$14
  Bottom 0.406: Q304.2 100.01,77.45 R304.2
N$15  (via drill 0.5)
  Top 0.406: v85.41,52.05 85.41,55.86 86.04,56.49 88.9,56.49 90.17,57.76 95.25,57.76 v96.84,56.18
  Bottom 0.406: IC201.9 v85.41,52.05 | v96.84,56.18 117.79,56.18 119.06,57.45 LED203.K
N$16
  Bottom 0.406: Q304.3 103.5,77.13 101.92,78.72 D318.C
N$17
  Bottom 0.406: RN301.7 71.75,78.4 74.61,81.26 84.14,81.26 86.68,78.72 D318.A
N$18
  Bottom 0.406: Q305.2 100.01,71.42 R305.2
N$19
  Bottom 0.406: Q305.3 103.5,71.1 101.92,72.69 D319.C
N$20
  Bottom 0.406: D319.A 71.12,72.69 RN302.1
N$21
  Bottom 0.406: Q306.2 100.01,65.39 R306.2
N$22
  Bottom 0.406: Q306.3 103.5,65.07 101.92,66.66 D320.C
N$23
  Bottom 0.406: RN302.3 71.12,67.29 72.39,68.56 86.36,68.56 D320.A
N$24
  Bottom 0.406: Q307.2 100.01,59.35 R307.2
N$25
  Bottom 0.406: Q307.3 103.5,59.03 101.92,60.62 D321.C
N$26
  Bottom 0.406: RN302.5 71.12,62.21 72.39,63.48 85.41,63.48 D321.A
N$27
  Bottom 0.406: Q301.2 100.01,95.55 R301.2
N$28
  Bottom 0.406: Q308.2 100.01,53.32 R308.2
N$29
  Bottom 0.406: Q308.3 103.5,53 101.92,54.59 D334.C
N$30
  Bottom 0.406: RN302.7 71.12,57.13 72.39,55.86 87,55.86 D334.A
N$31  (via drill 0.5)
  Top 0.406: v90.17,51.73 94.61,51.73 v96.2,50.14 | v118.75,50.78 118.75,59.67 LED211.K
  Bottom 0.406: IC201.10 86.04,54.59 87.31,53.32 88.58,53.32 v90.17,51.73 | v96.2,50.14 118.11,50.14 v118.75,50.78
N$32
  Bottom 0.406: Q309.2 100.01,47.29 R309.2
N$33
  Bottom 0.406: Q301.3 103.5,95.23 101.92,96.82 D315.C
N$34
  Bottom 0.406: Q309.3 103.5,46.97 101.92,48.56 D335.C
N$35
  Bottom 0.406: RN303.1 70.8,52.68 71.44,53.32 86.04,53.32 86.68,52.68 86.68,49.19 87.31,48.56 D335.A
N$36
  Bottom 0.406: Q310.2 100.01,41.25 R310.2
N$37
  Bottom 0.406: Q310.3 103.5,40.94 101.92,42.52 D336.C
N$38
  Bottom 0.406: RN301.1 78.11,93.64 78.74,93.01 84.45,93.01 D315.A
N$39
  Bottom 0.406: RN303.3 72.07,44.75 86.04,44.75 D336.A
N$40
  Bottom 0.406: Q311.2 100.01,35.22 R311.2
N$41
  Bottom 0.406: Q311.3 103.5,34.9 101.92,36.49 D337.C
N$42
  Bottom 0.406: RN303.5 71.12,40.94 72.39,39.67 85.09,39.67 D337.A
N$43
  Bottom 0.406: Q312.2 100.01,29.19 R312.2
N$44
  Bottom 0.406: Q312.3 103.5,28.87 101.92,30.46 D338.C
N$45  (via drill 0.5)
  Top 0.406: v84.77,34.59 86.68,32.68 86.68,30.78 87,30.46 D338.A
  Bottom 0.406: RN303.7 72.07,34.59 v84.77,34.59
N$46
  Bottom 0.406: Q313.2 100.01,23.16 R313.2
N$47
  Bottom 0.406: Q313.3 103.5,22.84 101.92,24.43 D339.C
N$48
  Bottom 0.406: RN304.1 72.07,29.82 72.39,29.51 85.72,29.51 86.68,28.55 86.68,26.02 D339.A
N$49  (via drill 0.5)
  Top 0.406: v78.74,38.4 80.01,39.67 85.09,39.67 86.68,38.08 103.82,38.08 v104.46,38.71 | LED205.K 120.33,40.3 119.7,40.94 119.7,44.75 v119.06,45.38 | v111.44,45.38 v111.44,42.21
  Bottom 0.406: IC202.4 v78.74,38.4 | v119.06,45.38 117.16,47.29 113.35,47.29 v111.44,45.38 | v111.44,42.21 110.17,40.94 105.09,40.94 104.78,40.62 104.78,39.03 v104.46,38.71
N$50  (via drill 0.5)
  Top 0.406: v77.47,62.21 77.47,70.78 78.42,71.73 v82.55,71.73 | v85.09,71.73 v85.09,92.37
  Bottom 0.406: IC201.4 v77.47,62.21 | v82.55,71.73 v85.09,71.73 | v85.09,92.37 120.97,92.37 LED201.K
N$51  (via drill 0.5)
  Top 0.406: LED209.K 119.7,87.93 v118.11,86.34 | v86.04,86.34 v86.04,60.94
  Bottom 0.406: v118.11,86.34 v86.04,86.34 | v86.04,60.94 77.15,60.94 75.88,59.67 IC201.5
N$52  (via drill 0.5)
  Top 0.406: LED202.K 120.65,82.85 v118.11,80.31
  Bottom 0.406: v118.11,80.31 91.12,80.31 90.17,79.36 90.17,59.67 89.53,59.03 87.63,59.03 87,58.4 77.15,58.4 75.88,57.13 IC201.6
N$53  (via drill 0.5)
  Top 0.406: LED210.K 121.28,77.77 v117.79,74.28 | v91.12,50.14 v85.41,50.14 | v77.47,48.56 v77.47,54.59
  Bottom 0.406: v117.79,74.28 91.76,74.28 91.12,73.64 v91.12,50.14 | v85.41,50.14 83.19,50.14 81.6,48.56 v77.47,48.56 | v77.47,54.59 IC201.7
N$54  (via drill 0.5)
  Top 0.406: v89.85,56.18 v93.03,56.18 | v93.03,62.21 v107,62.21 | v118.43,62.84 118.43,64.43 LED204.K
  Bottom 0.406: IC201.11 87,57.13 87.95,56.18 v89.85,56.18 | v93.03,56.18 v93.03,62.21 | v107,62.21 117.79,62.21 v118.43,62.84
N$55  (via drill 0.5)
  Top 0.406: v85.09,59.67 v85.09,69.83 | v88.9,68.24 v107.31,68.24 | v118.43,69.2 118.43,71.1 120.02,72.69 LED212.K
  Bottom 0.406: IC201.12 v85.09,59.67 | v85.09,69.83 86.36,69.83 87.95,68.24 v88.9,68.24 | v107.31,68.24 117.47,68.24 v118.43,69.2
N$56  (via drill 0.5)
  Top 0.406: LED207.K 121.28,4.74 118.11,7.92 v116.2,7.92 | v82.87,16.17 82.87,27.92 82.55,28.24 IC202.9
  Bottom 0.406: v116.2,7.92 86.36,7.92 84.14,10.14 84.14,14.9 v82.87,16.17
N$57  (via drill 0.5)
  Top 0.406: LED213.K 120.97,35.22 119.7,36.49 119.7,38.4 118.43,39.67 118.43,43.16 117.47,44.11 v116.2,44.11 | v77.47,42.21 v77.47,35.86
  Bottom 0.406: v116.2,44.11 93.66,44.11 90.49,40.94 85.41,40.94 84.14,42.21 v77.47,42.21 | v77.47,35.86 IC202.5
N$58  (via drill 0.5)
  Top 0.406: v79.38,33.32 v79.38,37.13 | v117.79,38.08 118.11,38.08 118.75,37.45 118.75,33 LED206.K
  Bottom 0.406: IC202.6 v79.38,33.32 | v79.38,37.13 84.14,37.13 86.36,34.9 93.03,34.9 96.2,38.08 103.5,38.08 103.82,37.76 105.09,37.76 105.41,38.08 v117.79,38.08
N$59  (via drill 0.5)
  Top 0.406: LED214.K 120.65,25.06 119.38,26.33 119.38,28.24 118.43,29.19 118.43,31.41 117.79,32.05 v116.2,32.05
  Bottom 0.406: v116.2,32.05 78.11,32.05 76.83,30.78 IC202.7
N$60  (via drill 0.5)
  Top 0.406: LED215.K 117.47,13.95 v116.2,13.95 | v83.82,18.08 83.82,30.14 83.19,30.78 IC202.10
  Bottom 0.406: v116.2,13.95 87.95,13.95 v83.82,18.08
N$61  (via drill 0.5)
  Top 0.406: LED208.K 120.02,14.9 119.38,15.54 119.38,18.39 117.79,19.98 v116.2,19.98 | v88.58,19.98 85.09,19.98 84.77,20.3 84.77,31.73 83.19,33.32 IC202.11
  Bottom 0.406: v116.2,19.98 v88.58,19.98
N$62  (via drill 0.5)
  Top 0.406: LED216.K 120.33,19.98 118.75,21.57 118.75,25.06 117.79,26.02 v116.2,26.02 | v88.58,26.02 86.36,26.02 85.72,26.65 85.72,31.73 83.82,33.63 83.82,35.22 83.19,35.86 IC202.12
  Bottom 0.406: v116.2,26.02 v88.58,26.02
N$63
  Bottom 0.406: Q314.2 100.01,17.12 R314.2
N$64
  Bottom 0.406: Q314.3 103.5,16.81 101.92,18.39 D346.C
N$65
  Bottom 0.406: RN304.3 72.07,24.75 73.34,26.02 83.82,26.02 86.36,23.48 86.36,20.3 D346.A
N$66
  Bottom 0.406: Q315.2 100.01,11.09 R315.2
N$67
  Bottom 0.406: Q315.3 103.5,10.78 101.92,12.36 D347.C
N$68
  Bottom 0.406: RN304.5 72.71,19.66 74.3,18.08 82.55,18.08 D347.A
N$69
  Bottom 0.406: Q316.2 100.01,5.06 R316.2
N$70
  Bottom 0.406: Q316.3 103.5,4.74 101.92,6.33 D348.C
N$71
  Bottom 0.406: RN304.7 72.39,14.59 74.3,16.49 81.28,16.49 83.19,14.59 83.19,9.51 86.36,6.33 D348.A
OUT1
  Top 0.406: D308.C 105.73,93.96 104.14,95.55 103.19,95.55 101.92,94.28 101.28,94.28 100.01,95.55 89.85,95.55 R301.1
  Bottom 0.813: X302.1 127.95,95.55 126.68,96.82 D301.A 112.39,96.82 109.54,93.96 D308.C
OUT2
  Top 0.406: D309.C 105.73,87.93 104.14,89.52 103.19,89.52 101.92,88.25 101.28,88.25 100.01,89.52 89.85,89.52 R302.1
  Bottom 0.813: X302.2 127.95,90.47 124.14,86.66 120.02,86.66 118.75,87.93 118.75,88.56 D302.A 112.39,90.79 109.54,87.93 D309.C
OUT3
  Top 0.406: D310.C 105.73,81.9 104.14,83.48 103.19,83.48 101.92,82.21 101.28,82.21 100.01,83.48 89.85,83.48 R303.1
  Bottom 0.813: X302.3 127.95,85.39 124.14,81.58 119.7,81.58 D303.A 112.39,84.75 109.54,81.9 D310.C
OUT4
  Top 0.406: D311.C 105.73,75.86 104.14,77.45 103.19,77.45 101.92,76.18 101.28,76.18 100.01,77.45 89.85,77.45 R304.1
  Bottom 0.813: X302.4 127.95,80.31 124.14,76.5 118.75,76.5 D304.A 112.39,78.72 109.54,75.86 D311.C
OUT5
  Top 0.406: D312.C 105.73,69.83 104.14,71.42 103.19,71.42 101.92,70.15 101.28,70.15 100.01,71.42 89.85,71.42 R305.1
  Bottom 0.813: X302.5 127.95,75.23 124.14,71.42 117.79,71.42 D305.A 112.39,72.69 109.54,69.83 D312.C
OUT6
  Top 0.406: D313.C 105.73,63.8 104.14,65.39 103.19,65.39 101.92,64.12 101.28,64.12 100.01,65.39 89.85,65.39 R306.1
  Bottom 0.813: X302.6 127.95,70.15 124.14,66.34 116.84,66.34 D306.A 112.39,66.66 109.54,63.8 D313.C
OUT7
  Top 0.406: D314.C 105.73,57.76 104.14,59.35 103.19,59.35 101.92,58.08 101.28,58.08 100.01,59.35 89.85,59.35 R307.1
  Bottom 0.813: X302.7 127.64,65.07 123.83,61.26 117.16,61.26 D307.A 112.08,60.62 109.22,57.76 D314.C
OUT8
  Top 0.406: D328.C 106.05,51.73 104.46,53.32 103.19,53.32 101.92,52.05 101.28,52.05 100.01,53.32 89.85,53.32 R308.1
  Bottom 0.813: X302.8 127,59.99 121.6,54.59 D322.A 112.08,54.59 109.22,51.73 D328.C
OUT9
  Top 0.406: D329.C 105.73,45.7 104.14,47.29 103.19,47.29 101.92,46.02 101.28,46.02 100.01,47.29 89.85,47.29 R309.1
  Bottom 0.813: X303.1 127,40.3 118.75,48.56 D323.A 112.08,48.56 109.22,45.7 D329.C
OUT10
  Top 0.406: D330.C 105.73,39.67 104.14,41.25 103.19,41.25 101.92,39.98 101.28,39.98 100.01,41.25 89.85,41.25 R310.1
  Bottom 0.813: X303.2 127.95,35.22 124.14,39.03 120.02,39.03 D324.A 114.62,42.52 111.76,39.67 D330.C
OUT11
  Top 0.406: D331.C 106.05,33.63 104.46,35.22 103.19,35.22 101.92,33.95 101.28,33.95 100.01,35.22 89.85,35.22 R311.1
  Bottom 0.813: X303.3 127.95,30.14 124.14,33.95 119.06,33.95 D325.A 112.08,36.49 109.22,33.63 D331.C
OUT12
  Top 0.406: D332.C 105.73,27.6 104.14,29.19 103.19,29.19 101.92,27.92 101.28,27.92 100.01,29.19 89.85,29.19 R312.1
  Bottom 0.813: X303.4 127.95,25.06 124.14,28.87 118.11,28.87 D326.A 112.08,30.46 109.22,27.6 D332.C
OUT13
  Top 0.406: D333.C 105.73,21.57 104.14,23.16 103.19,23.16 101.92,21.89 101.28,21.89 100.01,23.16 89.85,23.16 R313.1
  Bottom 0.813: X303.5 127.95,19.98 124.14,23.79 117.16,23.79 D327.A 112.39,24.43 109.54,21.57 D333.C
OUT14
  Top 0.406: D343.C 105.73,15.54 104.14,17.12 103.19,17.12 101.92,15.86 101.28,15.86 100.01,17.12 89.85,17.12 R314.1
  Bottom 0.813: X303.6 127.95,14.9 124.14,18.71 116.84,18.71 D340.A 112.39,18.39 109.54,15.54 D343.C
OUT15
  Top 0.406: D344.C 105.73,9.51 104.14,11.09 103.19,11.09 101.92,9.82 101.28,9.82 100.01,11.09 89.85,11.09 R315.1
  Bottom 0.813: X303.7 127.95,9.82 124.14,13.63 117.79,13.63 D341.A 111.76,12.36 108.9,9.51 D344.C
OUT16
  Top 0.406: D345.C 105.73,3.47 104.14,5.06 103.19,5.06 101.92,3.79 101.28,3.79 100.01,5.06 89.85,5.06 R316.1
  Bottom 0.813: X303.8 127.95,4.74 124.14,8.55 118.75,8.55 D342.A 111.76,6.33 108.9,3.47 D345.C
PLUGGED  (via drill 0.5)
  Top 0.406: v13.34,76.5 v13.34,73.01 | v40.01,73.96 IC101.39
  Bottom 0.406: CON101.3 10.65,79.18 v13.34,76.5 | v13.34,73.01 31.11,73.01 31.43,72.69 38.73,72.69 v40.01,73.96
Q-CLK
  Top 0.61: IC101.13 33.02,46.02 30.8,43.79 30.8,28.24 | 30.8,28.24 QG101.8 | 30.8,28.24 30.8,27.6 32.38,26.02 34.29,26.02 35.24,25.06 IC104.8
SCK  (via drill 0.5)
  Top 0.406: IC103.6 50.48,7.6 49.21,8.87 45.72,8.87 44.13,10.46 38.42,10.46 38.1,10.14 SV101.3 | IC104.13 40.32,19.66 41.59,20.93 41.59,24.75 37.47,28.87 v37.47,58.72
  Bottom 0.406: SV101.3 38.1,11.09 40.32,13.32 IC104.13 | v37.47,58.72 IC101.8
SCL  (via drill 0.5)
  Top 0.406: IC202.14 79.69,40.94 78.74,41.89 v78.74,47.29 v78.74,64.75
  Bottom 0.406: IC101.22 52.39,30.78 53.66,29.51 R201.1 56.2,28.55 64.45,28.55 65.09,29.19 65.09,46.65 65.72,47.29 v78.74,47.29 | v78.74,64.75 IC201.14
SDA  (via drill 0.5)
  Top 0.406: v79.69,43.48 v79.69,49.83 79.69,66.66 80.33,67.29 IC201.15
  Bottom 0.406: IC101.23 R202.1 53.66,31.73 62.87,31.73 64.14,33 64.14,48.24 65.72,49.83 v79.69,49.83 | IC202.15 v79.69,43.48
SPG
  Bottom 0.61: R106.2 R107.1 44.77,78.72 46.99,76.5 IC101.40
V+
  Top 0.813: OK201.7 65.72,91.1 65.09,90.47 65.09,86.02 | 65.09,86.02 65.09,80.94 | 65.09,80.94 65.09,75.86 | 65.09,75.86 65.09,69.83 | 65.09,69.83 65.09,64.75 | 65.09,64.75 65.09,59.67 | 65.09,59.67 65.09,54.59 | 65.09,54.59 65.09,48.56 | 65.09,48.56 65.09,43.48 | 65.09,43.48 65.09,38.08 | 65.09,38.08 65.09,33.32 | 65.09,33.32 65.09,27.29 | 65.09,27.29 65.09,22.21 | 65.09,22.21 65.09,16.81 | 65.09,16.81 65.09,12.04 | 65.09,12.04 65.09,9.82 65.72,9.19 74.3,9.19 75.88,7.6 DC201.4 | 65.09,12.04 OK204.1 | OK204.3 65.41,17.12 65.09,16.81 | 65.09,22.21 OK204.5 | 65.09,27.29 OK204.7 | OK203.3 65.41,38.4 65.09,38.08 | 65.09,43.48 OK203.5 | 65.09,48.56 OK203.7 | 65.09,59.67 OK202.3 | 65.09,64.75 OK202.5 | 65.09,69.83 OK202.7 | 65.09,75.86 OK201.1 | 65.09,80.94 OK201.3 | 65.09,86.02 OK201.5 | 65.09,54.59 OK202.1 | 65.09,33.32 OK203.1
  Bottom 0.813: C201.1 76.83,12.04 75.88,11.09 DC201.4
V-NETZTEIL1
  Bottom 1.27: CON101.1 19.05,90.47 21.91,93.33 D103.A

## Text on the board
tNames: HW: 23.11.25 | 1 | 2 | +18V | DC | 3 | Status | 4 | 5 | 6 | (c) Dr.-Ing. Th. Wiesner | MBCAN-Projekt | 7 | 8 | 0 | Booster | B | 9 | IN | 10 | 11 | 12 | 13 | OUT | 14 | 15 | 16 | mbc-90-DC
